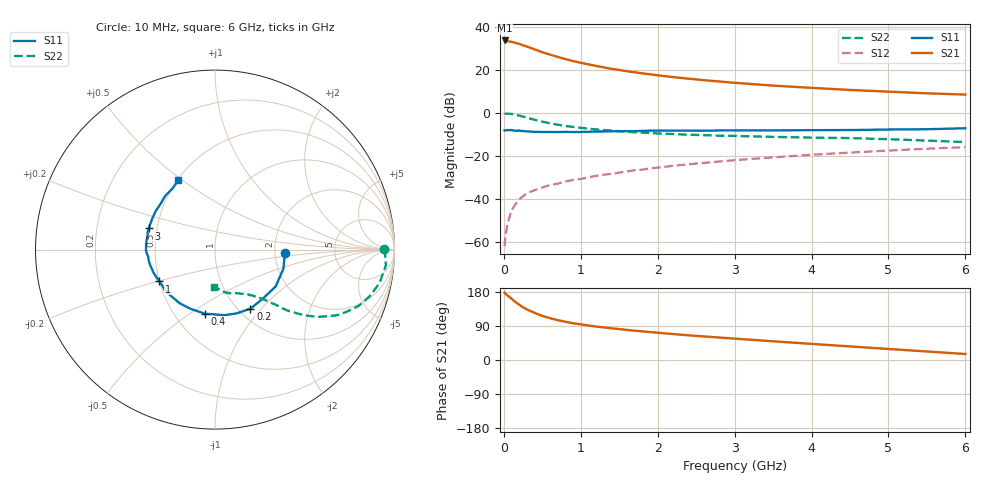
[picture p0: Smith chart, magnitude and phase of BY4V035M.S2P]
! SIEMENS Small Signal Semiconductors
! BFY420
! Si NPN RF SIEGET Grounded Emitter Transistor in MICRO-X
! VCE = 4 V  IC = 35 mA
! Common Emitter S-Parameters:  October  1996
# GHz  S  MA  R  50
!  f  S11  S21  S12  S22
! GHz  MAG  ANG  MAG  ANG  MAG  ANG  MAG  ANG
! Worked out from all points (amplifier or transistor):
!   36 points, 10 MHz to 6 GHz, reference 50 ohm
!   highest |S21| = 33.6 dB at 10 MHz (marker M1)
!   |S21| within 3 dB of that: start of sweep to 311.9 MHz
!   unconditionally stable (mu >= 1): start of sweep to 12.42 MHz; 1.616 GHz to end of sweep
!   at 250 MHz: K = 0.39, MSG = 35.1 dB, |S12| = -38.8 dB
!   at 1.4 GHz: K = 0.97, MSG = 24.4 dB, |S12| = -28.4 dB
!   at 6 GHz: K = 1.05, MAG = 10.9 dB, |S12| = -16.0 dB
!   S11 on the Smith chart (normalised r, x): 10 MHz: 2.28, -0.10; 200 MHz: 1.13, -0.88; 400 MHz: 0.70, -0.57; 1 GHz: 0.50, -0.20; 3 GHz: 0.45, +0.12; 6 GHz: 0.51, +0.48
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0.01  0.3908 -2.6  47.63 177.8  0.0008 112.6  0.9428 0.2
0.02  0.3895 -6.0  47.28 174.8  0.0014 70.6  0.9475 -1.2
0.1  0.3957 -31.2  44.24 161.8  0.0055 79.0  0.936 -11.4
0.15  0.3817 -45.5  41.97 152.9  0.0075 73.1  0.8999 -16.8
0.2  0.384 -59.0  39.64 146.1  0.0098 70.8  0.8597 -21.4
0.25  0.3754 -71.2  36.91 139.0  0.0115 67.1  0.8111 -25.3
0.3  0.369 -82.1  34.33 133.4  0.0135 67.0  0.7688 -28.5
0.4  0.3613 -99.2  29.56 124.4  0.016 65.4  0.6868 -33.1
0.5  0.357 -113.0  25.4 116.2  0.0184 63.6  0.621 -36.2
0.6  0.358 -123.7  22.34 110.4  0.0209 63.6  0.5698 -38.2
0.7  0.3555 -132.1  19.82 105.1  0.0226 63.7  0.529 -40.0
0.9  0.3557 -144.8  15.85 97.0  0.0275 63.0  0.468 -41.8
1  0.3575 -150.3  14.45 94.0  0.0291 64.1  0.4466 -42.7
1.1  0.3613 -155.5  13.29 91.0  0.0316 64.1  0.4273 -43.8
1.3  0.3671 -162.5  11.28 85.9  0.0365 64.5  0.3964 -45.1
1.6  0.3745 -171.7  9.201 79.3  0.0435 64.2  0.3617 -47.6
2.2  0.3847 175.5  6.713 68.5  0.0586 62.2  0.3209 -52.3
3  0.3876 162.3  4.957 56.4  0.0792 57.4  0.2899 -58.4
3.5  0.3896 154.2  4.264 49.4  0.0923 53.8  0.2749 -62.3
4.5  0.3966 139.5  3.382 35.8  0.1188 45.8  0.258 -70.9
5.5  0.4147 124.8  2.823 22.5  0.1461 36.8  0.2255 -83.0
6  0.4367 117.9  2.64 15.8  0.1592 31.9  0.2084 -90.8
